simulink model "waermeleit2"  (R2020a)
settings: Solver=ode45  StartTime=0.0  StopTime=2000  MaxStep=20  RelTol=1e-3  EnableMultiTasking=on
InitFcn:
  | init_waermeleit2
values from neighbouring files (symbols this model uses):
  A = 0.1    [init_sink.m]    (also in init_waermeleit2.m = diag(-2*ones(N+1,1)) + diag(ones(N,1), 1) + diag(ones(N,1), )
  c1 = 1e7    (= 10000000)    [init_sink.m]    (also in init_waermeleit1.m = 0.002908; init_waermeleit2.m = 0.0727)
  N = 5    [init_waermeleit1.m]    (also in init_waermeleit2.m = 25; sfun_pendelanim.m = 24; solve_euler.m = ceil((t1 - t0)/h) + 1; solve_euler1d.m = ceil((t1 - t0)/h) + 1)
  T0 = 500    [init_waermeleit1.m]    (also in init_waermeleit2.m)
  Tl = 300    [init_waermeleit1.m]    (also in init_waermeleit2.m)
  Tr = 250    [init_waermeleit1.m]    (also in init_waermeleit2.m)

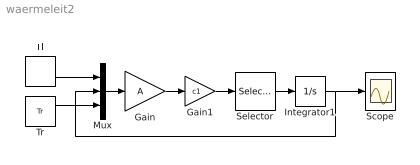
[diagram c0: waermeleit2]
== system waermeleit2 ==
  Gain : Gain  Gain=A  Multiplication=Matrix(K*u)
  Gain1 : Gain  Gain=c1
  Integrator1 : Integrator  InitialCondition=T0*ones(N-1,1)
  Mux : Mux  Inputs=3
  Scope : Scope
  Selector : Selector  InputPortWidth=N+1  IndexOptions=Index vector (dialog)  Indices=2:N  OutputSizes=1
  Tl : Constant  Value=Tl
  Tr : Constant  Value=Tr
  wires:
  Integrator1/1 -> Mux/2, Scope/1
  Tl/1 -> Mux/1
  Tr/1 -> Mux/3
  Mux/1 -> Gain/1
  Gain/1 -> Gain1/1
  Gain1/1 -> Selector/1
  Selector/1 -> Integrator1/1
